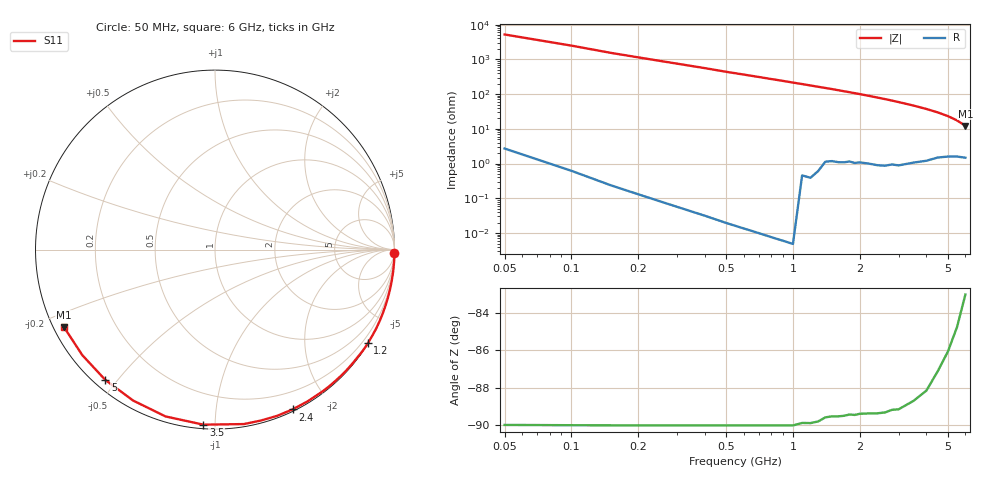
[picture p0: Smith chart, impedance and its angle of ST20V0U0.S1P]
! SIEMENS Discrete & RF Semiconductors
! BA892
! Si PIN Diode in SCD-80
! VR = 20 V
! S-Parameters:  September  1997
# GHz  S  MA  R  50
!  f  S11
! GHz  MAG  ANG
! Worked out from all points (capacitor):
!   34 points, 50 MHz to 6 GHz, reference 50 ohm
!   read as one part to ground: C = 639 fF near 50 MHz
!   lowest |Z| = 12.2 ohm at 6 GHz (marker M1)
!   S11 on the Smith chart (normalised r, x): 50 MHz: open; 1.2 GHz: 0.01, -3.55; 2.4 GHz: 0.02, -1.60; 3.5 GHz: 0.02, -0.94; 5 GHz: 0.03, -0.46; 6 GHz: 0.03, -0.24
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0.05  1 -1.1
0.1  1 -2.3
0.2  1 -5.0
0.4  1 -10.2
0.5  1 -13.0
0.6  1 -15.6
0.7  1 -18.2
0.8  1 -20.9
0.9  1 -23.5
1  1 -26.2
1.2  0.9989 -31.5
1.3  0.9979 -34.2
1.5  0.9947 -39.4
1.6  0.9943 -42.2
1.8  0.9925 -47.6
1.9  0.9925 -50.3
2  0.9914 -53.0
2.2  0.9905 -58.5
2.4  0.9899 -64.1
2.6  0.9888 -69.6
2.8  0.9861 -75.1
3  0.9853 -80.6
3.5  0.9775 -93.8
4  0.9695 -106.5
4.5  0.9568 -118.5
5  0.949 -130.1
5.5  0.9447 -141.5
6  0.9458 -152.8
